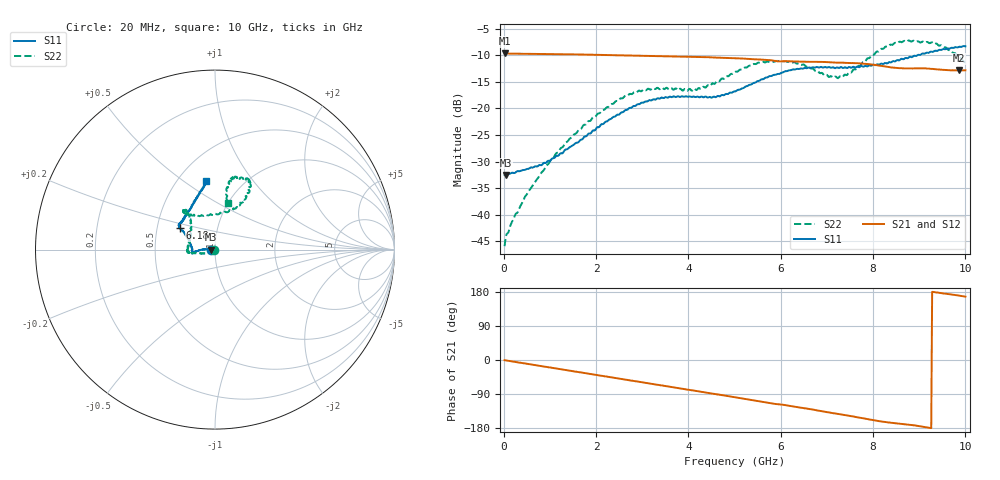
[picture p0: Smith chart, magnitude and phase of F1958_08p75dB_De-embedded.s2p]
! Integrated Device Technology
! Corporate Headquarters
! 6024 Silver Creek Valley Road
! San Jose, CA 95138  USA
! Phone:  1-408-284-8200
! Toll Free:  1-800-223-1366
! Webpage:  http://www.idt.com/
! Timing and RF Division
! 515 Groton Road, Suite 102
! Westford, MA 01886-6024
! Device:  F1958
! Description: 7-bit 0.25 dB Digital Step Attenuator
! Frequency:  0.001 -  6.000 GHz
! Package:  4x4 mm Thin QFN Plastic Package: 24 pin
! Ports:  2 RF, 12 DC
!  Pin  1  = D0
!  Pin  2  = VDD
!  Pin  3  = VMODE
!  Pin  4  = GND
!  Pin  5  = RF1  =  Port 1
!  Pin  6  = GND
!  Pin  7  = GND
!  Pin  8  = GND
!  Pin  9  = GND
!  Pin 10  = GND
!  Pin 11  = GND
!  Pin 12  = GND
!  Pin 13  = GND
!  Pin 14  = RF2  =  Port 2
!  Pin 15  = GND
!  Pin 16  = LE
!  Pin 17  = CLK
!  Pin 18  = DATA
!  Pin 19  = D6
!  Pin 20  = D5
!  Pin 21  = D4
!  Pin 22  = D3
!  Pin 23  = D2
!  Pin 24  = D1
! State:  35
! Atten State:  8.75 dB
! Voltage:  +3.30 Volts
! Current:  0.258 mA
! Data:  The device was measured on a F1958 evaluation board which has
!  individual transmission lines to the RF pins.  Data was collected
!  using a calibrated network analyzer.  The evaluation board was
!  de-embedded using Automatic Fixture Removal (AFR).
!  The reference plane is the edge of the package pin.
! Misc:
!  Action Tracker AT0419
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# GHz S dB R 50
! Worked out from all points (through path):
!   500 points, 20 MHz to 10 GHz, reference 50 ohm
!   highest |S21| = -9.65 dB at 20 MHz (marker M1); lowest = -12.9 dB at 9.86 GHz (marker M2)
!   group delay of S21, straight-line fit = 54.1 ps
!   lowest |S11| = -32.5 dB at 40 MHz (marker M3), VSWR 1.05, Z = 47.7 - j0.0739 ohm
!   |S11| at or under -10 dB: start of sweep to 8.958 GHz
!   |S22| runs from -45.9 to -7.2 dB; largest |S21 - S12| = 0.0009
!   S11 on the Smith chart (normalised r, x): 20 MHz: 0.95, -0.00; 6.18 GHz: 0.66, +0.16; 10 GHz: 0.68, +0.61
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0.02  -32.50 -178.1  -9.65 -0.5  -9.65 -0.5  -45.94 -156.2
0.04  -32.54 -178.1  -9.66 -0.9  -9.66 -0.9  -44.49 -150.1
0.22  -32.17 178.4  -9.69 -4.5  -9.69 -4.5  -40.72 -143.9
0.68  -30.91 175.0  -9.73 -13.5  -9.73 -13.5  -33.86 -142.3
1.14  -28.94 176.7  -9.77 -22.6  -9.77 -22.6  -28.43 -149.2
1.7  -25.83 178.5  -9.85 -33.5  -9.84 -33.4  -23.54 -161.6
2.58  -20.71 -175.8  -10.01 -50.7  -10.00 -50.7  -18.07 -171.0
3.36  -18.15 -171.5  -10.17 -65.9  -10.17 -66.0  -16.30 -176.3
4.22  -17.85 -175.1  -10.31 -82.8  -10.32 -82.8  -16.16 155.0
4.56  -17.78 178.3  -10.42 -89.5  -10.43 -89.5  -15.39 141.8
5.02  -16.79 164.5  -10.54 -98.6  -10.55 -98.6  -13.08 129.1
5.54  -14.78 153.6  -10.79 -108.8  -10.80 -108.8  -11.42 126.7
6.18  -12.83 148.7  -11.12 -120.8  -11.14 -120.7  -11.19 129.4
6.68  -12.28 145.7  -11.22 -130.5  -11.24 -130.4  -12.47 124.3
7.06  -12.23 142.7  -11.30 -138.8  -11.31 -138.7  -14.05 106.3
7.3  -12.23 140.0  -11.38 -143.5  -11.38 -143.4  -13.97 89.2
7.9  -11.97 128.7  -11.65 -156.5  -11.64 -156.6  -10.54 61.7
8.34  -11.32 119.2  -12.21 -164.9  -12.21 -165.0  -8.25 59.6
8.76  -10.50 110.5  -12.48 -170.5  -12.49 -170.4  -7.24 64.6
9.26  -9.31 102.9  -12.56 -179.7  -12.55 -179.8  -7.57 74.7
9.86  -8.41 97.9  -12.85 170.0  -12.88 170.1  -10.28 77.1
10  -8.30 97.8  -12.82 167.2  -12.85 167.3  -11.47 74.6
